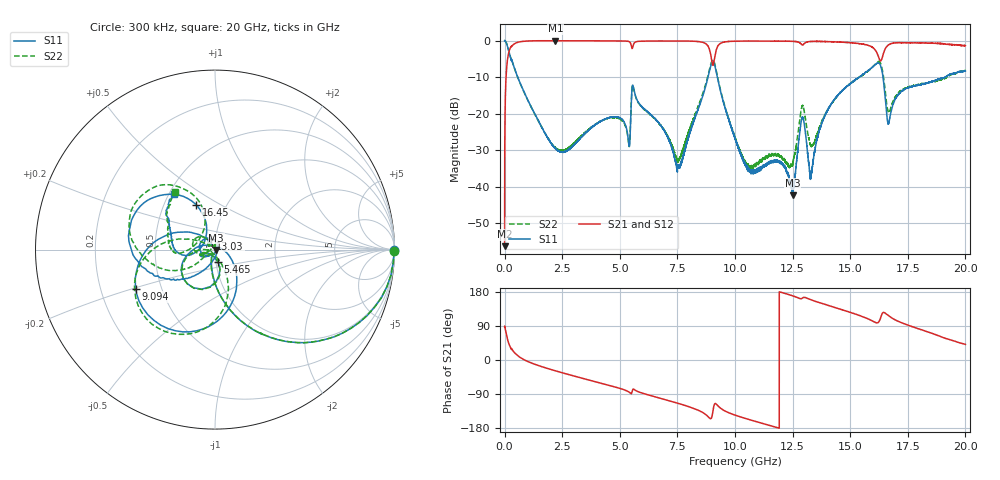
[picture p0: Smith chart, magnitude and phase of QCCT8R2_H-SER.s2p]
!{QCCT8R2}
!Johanson Technology Inc.
!www.johansontechnology.com
!Test Board Conditions:
!Substrate Type  RO4350B
!Substrate Thickness  20 mil
!Substrate Dk  3.66
!TL Type: GCPW
!TL Trace Width  34 mil
!TL Gap  10 mil
!Electrode orientation  Horizontal
!DUT TOPOLOGY	SERIES
!Mounting Pad LxW  26x52 mil
# MHz S  dB  R 50
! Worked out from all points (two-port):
!   20001 points, 300 kHz to 20 GHz, reference 50 ohm
!   highest |S21| = -0.03 dB at 2.208 GHz (marker M1); lowest = -56.3 dB at 300 kHz (marker M2)
!   |S21| within 3 dB of the highest: 190.1 MHz to 8.919 GHz (8.729 GHz wide, 192 % of centre); 9.165 GHz to 16.13 GHz (6.967 GHz wide, 55.1 % of centre)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
!   lowest |S11| = -42.4 dB at 12.5 GHz (marker M3), VSWR 1.02, Z = 50.7 - j0.262 ohm
!   |S11| at or under -10 dB: 567.8 MHz to 8.829 GHz (8.261 GHz wide, 176 % of centre); 9.235 GHz to 15.39 GHz (6.151 GHz wide, 50 % of centre); 16.42 GHz to 19.13 GHz (2.703 GHz wide, 15.2 % of centre)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
!   |S22| runs from -35.1 to 0.0 dB; largest |S21 - S12| = 0.017
!   S11 on the Smith chart (normalised r, x): 300 kHz: open; 5.465 GHz: 1.02, -0.14; 9.094 GHz: 0.36, -0.21; 13.03 GHz: 0.95, +0.12; 16.45 GHz: 0.72, +0.39; 20 GHz: 0.53, +0.39
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0.3  -0.02 -0.3  -56.27 87.1  -55.81 89.8  -0.02 -0.4
106.298  -1.20 -30.6  -6.25 59.2  -6.23 59.1  -1.19 -30.6
241.296  -4.26 -55.0  -2.11 34.6  -2.11 34.5  -4.25 -54.9
2208.267  -29.58 -117.4  -0.03 -28.6  -0.04 -28.6  -29.33 -123.5
3334.25  -26.41 -134.8  -0.05 -47.5  -0.05 -47.5  -26.11 -142.7
5465.218  -22.98 -76.8  -0.71 -87.9  -0.72 -87.9  -22.55 -75.9
5609.216  -13.34 -150.6  -0.85 -77.3  -0.85 -77.3  -13.38 -149.5
6667.2  -22.34 162.7  -0.11 -99.5  -0.12 -99.4  -22.34 -179.9
7568.186  -34.61 75.6  -0.11 -115.1  -0.11 -115.1  -32.38 -118.4
8756.169  -11.81 -62.9  -0.99 -145.3  -0.98 -145.2  -11.31 -75.4
9094.164  -6.14 -153.6  -5.50 -118.6  -5.46 -118.8  -5.83 -150.6
10000.15  -26.79 124.0  -0.17 -145.4  -0.17 -145.4  -26.47 140.9
10593.14  -35.00 128.8  -0.13 -156.7  -0.14 -156.8  -34.37 105.1
12496.11  -42.37 -19.8  -0.21 169.4  -0.21 169.4  -33.96 166.7
12868.11  -22.35 -165.9  -0.92 161.6  -0.92 161.7  -19.14 -174.0
13025.1  -23.70 110.7  -0.74 165.2  -0.73 165.3  -20.20 133.7
13334.1  -35.46 -38.9  -0.23 158.1  -0.24 158.1  -28.86 165.5
14416.08  -15.30 -125.8  -0.40 137.0  -0.36 137.0  -15.41 -145.0
16136.06  -6.34 173.9  -3.06 98.2  -3.09 98.3  -6.13 165.5
16451.05  -11.39 112.8  -3.37 125.5  -3.42 126.1  -10.15 110.2
16667.05  -22.68 159.8  -1.14 116.7  -1.23 116.9  -19.61 145.3
20000  -8.36 126.3  -1.39 41.1  -1.47 40.9  -8.18 124.6
